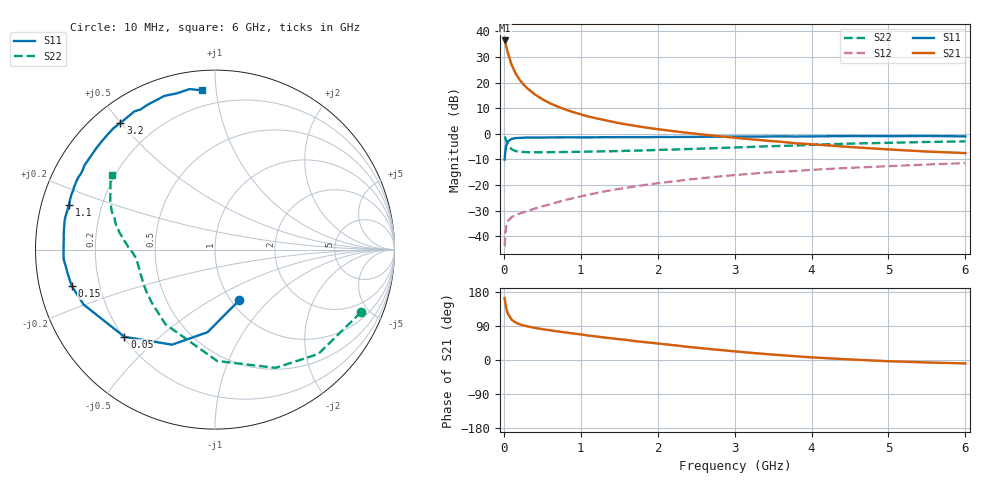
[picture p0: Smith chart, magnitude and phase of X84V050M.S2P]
! SIEMENS Small Signal Semiconductors
! BFP136W
! Si NPN RF Bipolar Junction Transistor in SOT343
! VCE = 4 V  IC = 50 mA
! Common Emitter S-Parameters:  September  1994
# GHz  S  MA  R  50
!  f  S11  S21  S12  S22
! GHz  MAG  ANG  MAG  ANG  MAG  ANG  MAG  ANG
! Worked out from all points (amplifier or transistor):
!   40 points, 10 MHz to 6 GHz, reference 50 ohm
!   highest |S21| = 36.4 dB at 10 MHz (marker M1)
!   |S21| within 3 dB of that: start of sweep to 37.16 MHz
!   unconditionally stable (mu >= 1): 681.3 MHz to 2.846 GHz
!   at 200 MHz: K = 0.54, MSG = 26.2 dB, |S12| = -31.2 dB
!   at 1.5 GHz: K = 1.10, MAG = 10.9 dB, |S12| = -21.5 dB
!   at 6 GHz: K = 0.96, MSG = 2.0 dB, |S12| = -11.5 dB
!   S11 on the Smith chart (normalised r, x): 10 MHz: 1.09, -0.68; 50 MHz: 0.20, -0.39; 150 MHz: 0.10, -0.12; 1.1 GHz: 0.08, +0.15; 3.2 GHz: 0.08, +0.50; 6 GHz: 0.11, +0.92
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0.01  0.313 -64.3  66.31 163.6  0.0064 72.7  0.8849 -23.2
0.02  0.4622 -95.2  59.13 149.1  0.0115 62.3  0.8184 -45.3
0.03  0.5811 -114.3  52.06 138.0  0.0151 53.3  0.7402 -62.9
0.05  0.7007 -136.1  39 123.1  0.0197 41.4  0.6207 -88.9
0.1  0.7935 -157.3  22.38 106.6  0.0236 32.8  0.4991 -123.6
0.15  0.8235 -165.7  15.38 99.3  0.0255 32.9  0.4602 -139.8
0.2  0.8311 -170.5  11.61 94.7  0.0276 34.3  0.4475 -149.0
0.25  0.8379 -174.0  9.379 91.5  0.0292 36.0  0.4417 -154.9
0.3  0.8451 -176.4  7.848 89.1  0.0308 38.0  0.4373 -158.8
0.4  0.8438 179.2  5.916 84.8  0.0346 41.8  0.4363 -164.1
0.5  0.8446 176.1  4.722 81.3  0.0383 45.2  0.4365 -167.5
0.6  0.8477 174.0  3.937 78.6  0.0421 47.8  0.4375 -169.6
0.7  0.85 171.2  3.395 75.4  0.0464 50.4  0.4389 -171.1
0.9  0.8532 167.5  2.654 70.0  0.0553 53.0  0.4428 -173.7
1.1  0.8508 162.9  2.171 64.4  0.0647 55.2  0.4485 -175.3
1.5  0.8589 156.1  1.613 55.0  0.0839 56.3  0.4602 -178.1
1.8  0.8587 150.6  1.357 47.8  0.0986 55.5  0.4723 179.7
2.2  0.8655 143.7  1.126 39.2  0.1176 53.6  0.4918 176.8
3.2  0.8814 126.7  0.784 19.2  0.1649 45.8  0.5529 167.9
4.5  0.9015 108.3  0.552 1.4  0.2166 34.2  0.6428 155.2
5.5  0.9056 99.0  0.45 -6.5  0.2508 26.4  0.6917 147.4
6  0.89 94.7  0.42 -9.0  0.2676 22.1  0.71 144.1
